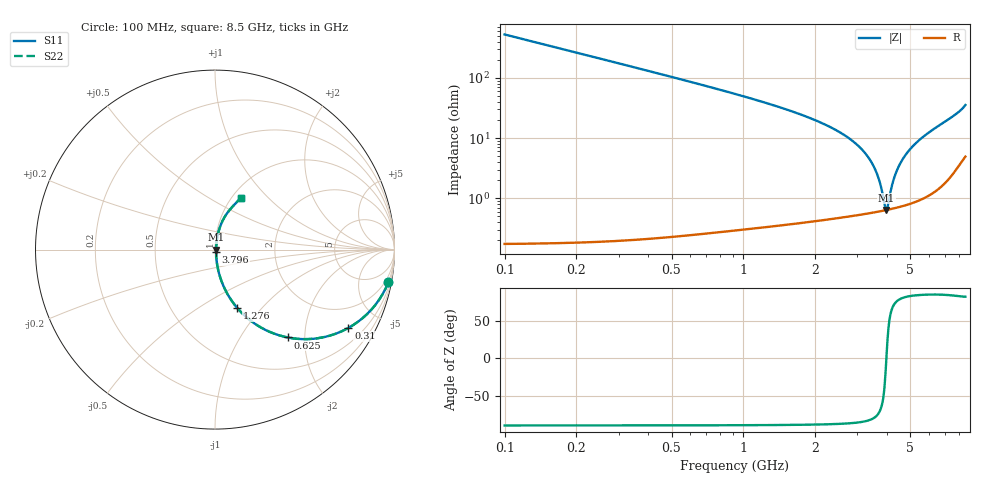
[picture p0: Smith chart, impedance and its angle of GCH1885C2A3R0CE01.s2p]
!Murata Part Number: GCH1885C2A3R0CE01
!These Parameters are Measured in Series Mode Connection
!Data Generated on Mar 13, 2026
!  o--ll--o
!Port1  Port2
!  o------o
!Operation Temp=25[degC], DC Bias Voltage=0[V]
!Freq. Start=100[MHz] Stop=9[GHz] 401[Steps]
# Hz S RI R 50
!Freq.(Hz) S11(Real) S11(Imag) S21(Real) S21(Imag) S12(Real) S12(Imag) S22(Real) S22(Imag)
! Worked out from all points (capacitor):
!   401 points, 100 MHz to 8.5 GHz, reference 50 ohm
!   read as one part in series: C = 3 pF near 142 MHz
!   lowest |Z| = 636 mohm at 3.964 GHz (marker M1)
!   series resonance near 3.968 GHz, so ESL is about 540 pH
!   S11 on the Smith chart (normalised r, x): 100 MHz: 1, -11; 310 MHz: 1.00, -3.40; 625 MHz: 1.00, -1.65; 1.276 GHz: 1.01, -0.75; 3.796 GHz: 1.01, -0.02; 8.5 GHz: 1.10, +0.70
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1e8  0.9656 -0.1821  0.0344 0.1821  0.0344 0.1821  0.9656 -0.1821
2.05e8  0.8693 -0.3367  0.1307 0.3367  0.1307 0.3367  0.8693 -0.3367
3.1e8  0.7428 -0.4365  0.2572 0.4365  0.2572 0.4365  0.7428 -0.4365
4.57e8  0.5672 -0.4945  0.4328 0.4945  0.4328 0.4945  0.5672 -0.4945
6.25e8  0.4066 -0.4897  0.5934 0.4897  0.5934 0.4897  0.4066 -0.4897
9.19e8  0.2309 -0.4188  0.7691 0.4188  0.7691 0.4188  0.2309 -0.4188
1.276e9  0.1242 -0.3254  0.8758 0.3254  0.8758 0.3254  0.1242 -0.3254
1.507e9  0.0861 -0.2745  0.9139 0.2745  0.9139 0.2745  0.0861 -0.2745
2.914e9  0.0121 -0.0833  0.9879 0.0833  0.9879 0.0833  0.0121 -0.0833
3.46e9  0.00707 -0.0369  0.9929 0.0369  0.9929 0.0369  0.00707 -0.0369
3.649e9  0.00643 -0.0226  0.9936 0.0226  0.9936 0.0226  0.00643 -0.0226
3.796e9  0.00624 -0.012  0.9938 0.012  0.9938 0.012  0.00624 -0.012
3.901e9  0.00625 -0.00463  0.9938 0.00463  0.9938 0.00463  0.00625 -0.00463
3.964e9  0.00631 -0.000295  0.9937 0.000295  0.9937 0.000295  0.00631 -0.000295
4.006e9  0.00637 0.00256  0.9936 -0.00256  0.9936 -0.00256  0.00637 0.00256
4.174e9  0.00678 0.0137  0.9932 -0.0137  0.9932 -0.0137  0.00678 0.0137
4.3e9  0.00726 0.0219  0.9927 -0.0219  0.9927 -0.0219  0.00726 0.0219
4.531e9  0.00848 0.0364  0.9915 -0.0364  0.9915 -0.0364  0.00848 0.0364
4.825e9  0.0106 0.0541  0.9894 -0.0541  0.9894 -0.0541  0.0106 0.0541
5.707e9  0.021 0.1042  0.979 -0.1042  0.979 -0.1042  0.021 0.1042
7.114e9  0.0541 0.1824  0.9459 -0.1824  0.9459 -0.1824  0.0541 0.1824
8.5e9  0.1434 0.2875  0.8566 -0.2875  0.8566 -0.2875  0.1434 0.2875
